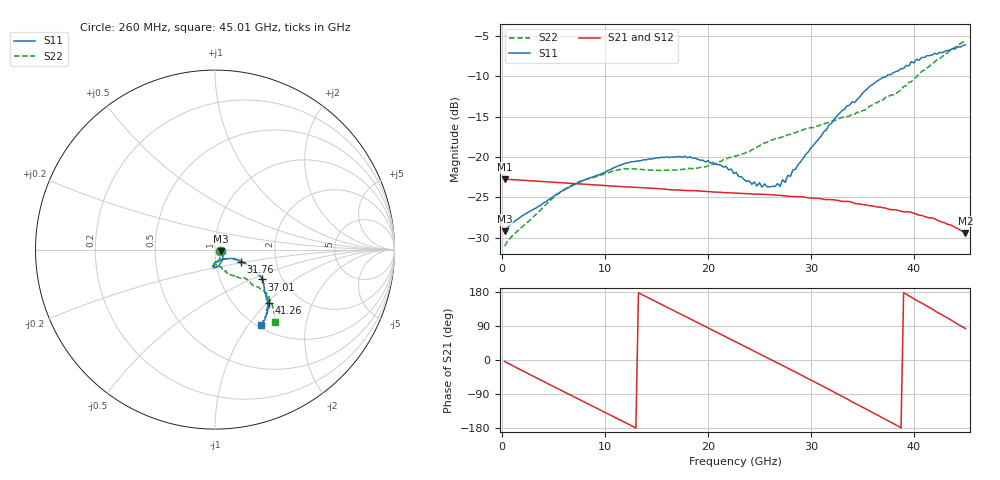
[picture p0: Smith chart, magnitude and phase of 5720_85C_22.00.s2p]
! Device:  ADRF5720
! Description: 0.5dB LSB GaAs MMIC 6-bit Digital Attenuator
! Frequency:  0.000009 -  40 GHz
! Ports:
!	RF1	= Port 1
!	RF2	= Port 2
! Vdd:  3.3 Volt
! Vss:  -3.3 Volt
! Control:  0/3.3 Volt
! State:  22.00 dB attenuation
! Data:  The device was measured using G-S-G Probes on a matrix board.
!  Data was collected using an calibrated 4 port network analyzer.
!  The reference plane for this measurement is at the launchers.
! Note:  Analog Devices supplies this data as a sample of measured data
!  for this product.  Your particular data for this product may vary.
!  Data was taken at 85 degrees C.
!  Analog Devices reserves the right to change this data at anytime.
# GHZ S DB R 45.0
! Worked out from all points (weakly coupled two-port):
!   180 points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, 260 MHz to 45.01 GHz, reference 45 ohm
!   highest |S21| = -22.75 dB at 260 MHz (marker M1); lowest = -29.4 dB at 45.01 GHz (marker M2)
!   lowest |S11| = -29.2 dB at 260 MHz (marker M3), VSWR 1.07, Z = 48.1 - j0.788 ohm
!   |S11| at or under -10 dB: start of sweep to 37.35 GHz
!   |S22| runs from -31.1 to -5.6 dB; largest |S21 - S12| = 0.00037
!   S11 on the Smith chart (normalised r, x): 260 MHz: 1.07, -0.02; 31.76 GHz: 1.32, -0.18; 37.01 GHz: 1.58, -0.58; 41.26 GHz: 1.42, -1.03; 45.01 GHz: 1.04, -1.16
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0.26  -29.23 -13.7  -22.75 -3.9  -22.74 -3.8  -31.05 -17.5
1.26  -27.92 -3.9  -22.84 -18.1  -22.83 -18.1  -29.45 -12.0
5.01  -24.88 -38.2  -23.13 -70.0  -23.12 -69.9  -25.02 -61.7
7.76  -23.03 -55.1  -23.36 -107.6  -23.34 -107.5  -22.94 -78.2
11.51  -21.01 -74.2  -23.66 -158.8  -23.65 -158.6  -21.54 -91.9
15.26  -20.12 -87.3  -23.93 149.7  -23.91 149.8  -21.65 -93.5
18.26  -19.99 -94.3  -24.17 109.0  -24.16 109.1  -21.42 -87.0
22.76  -21.92 -91.6  -24.49 47.3  -24.47 47.5  -19.86 -72.5
24.26  -23.39 -84.8  -24.59 26.9  -24.58 27.1  -19.14 -69.2
27.01  -23.64 -53.6  -24.75 -11.2  -24.73 -10.9  -17.61 -64.1
27.26  -22.82 -48.6  -24.80 -14.8  -24.78 -14.5  -17.50 -64.5
27.51  -23.17 -47.3  -24.83 -18.1  -24.82 -17.9  -17.45 -63.5
27.76  -22.28 -42.5  -24.85 -21.5  -24.84 -21.2  -17.26 -64.1
28.01  -22.41 -42.4  -24.89 -25.1  -24.87 -24.8  -17.21 -63.4
30.26  -18.53 -27.3  -25.09 -56.3  -25.08 -56.0  -16.39 -61.4
31.76  -16.05 -25.1  -25.28 -77.2  -25.27 -76.9  -15.74 -59.2
33.51  -13.69 -25.7  -25.51 -102.5  -25.49 -102.1  -14.98 -54.6
37.01  -10.15 -32.3  -26.30 -153.3  -26.28 -152.9  -12.95 -44.5
37.76  -9.81 -33.8  -26.52 -164.1  -26.50 -163.8  -12.34 -43.3
41.26  -7.48 -44.9  -27.47 142.4  -27.45 142.8  -9.00 -40.4
43.51  -6.80 -50.5  -28.40 107.1  -28.38 107.5  -6.83 -45.0
45.01  -6.11 -58.5  -29.41 82.9  -29.38 83.1  -5.58 -50.4
